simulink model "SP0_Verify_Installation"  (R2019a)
settings: Solver=VariableStepAuto  StartTime=0.0  StopTime=0.01  FixedStep=1e-5  RelTol=5e-6
libraries: ee_lib x3, fl_lib x2, nesl_utility x2

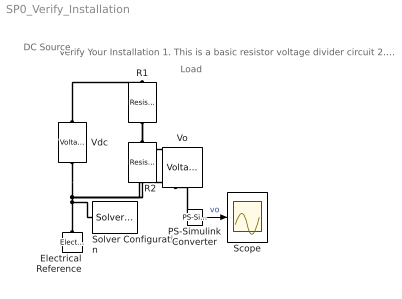
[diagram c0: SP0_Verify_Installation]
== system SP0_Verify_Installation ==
  note: Verify Your Installation 1. This is a basic resistor voltage divider circuit 2. Ensure you see a DC source and 2 resistors in the diagram 3. If you do not, you may have to re-install the Simscape Package 4. Simulate the circuit (click the Run button above) 5. Open the Scope below (double click) 6. Observe the voltage waveform 7. If you see a line at 5 V, your installation is correct, hurray! 8. If the simulation does not run, check with a classmate, TA, or Prof. Kim _________________________________
  note: Load
  note: DC Source
  Electrical Reference : fl_lib/Electrical/Electrical Elements/Electrical Reference
  PS-Simulink Converter : nesl_utility/PS-Simulink Converter  PhysicalDomain=network_engine_domain  SubClassName=ps_output  LeftPortType=input  RightPortType=output  PseudoPeriodic=off  Frequencies=[]  Unit=1  AffineConversion=off
  R1 : ee_lib/Passive/Resistor  R=5 Ohm  R_tol=1  enable_R_tol=0  tol_distribution=1  nSigma=4  enable_operating_limits=0  operating_limit_action=2  max_working_voltage=100 V  power_rating=1 W  enable_faults=0  fault_action=1  R_faulted=inf Ohm  enable_temporal_fault=0  t_fault=1 s  enable_behavioral_fault=0  max_permissible_current=1 A  t_fail_on_current=1 s  noise_mode=0  sample_time=1e-3 s  repeatability=1  auto_seed=1127352614  user_seed=0  Tdevice=25 degC  alpha=3.93e-3 1/K  Tmeas=25 degC  thermal_mass=100 J/K  power_derating_T1=70 degC  power_derating_T2=155 degC  operating_temperature_range_vec=[-50, 150] degC  temperature_specify=off  temperature_priority=High  temperature=298.15 K  temperature_nominal_specify=off  temperature_nominal_unit=K  temperature_nominal_value=1
  R2 : ee_lib/Passive/Resistor  R=5 Ohm  R_tol=1  enable_R_tol=0  tol_distribution=1  nSigma=4  enable_operating_limits=0  operating_limit_action=2  max_working_voltage=100 V  power_rating=1 W  enable_faults=0  fault_action=1  R_faulted=inf Ohm  enable_temporal_fault=0  t_fault=1 s  enable_behavioral_fault=0  max_permissible_current=1 A  t_fail_on_current=1 s  noise_mode=0  sample_time=1e-3 s  repeatability=1  auto_seed=529650792  user_seed=0  Tdevice=25 degC  alpha=3.93e-3 1/K  Tmeas=25 degC  thermal_mass=100 J/K  power_derating_T1=70 degC  power_derating_T2=155 degC  operating_temperature_range_vec=[-50, 150] degC  temperature_specify=off  temperature_priority=High  temperature=298.15 K  temperature_nominal_specify=off  temperature_nominal_unit=K  temperature_nominal_value=1
  Scope : Scope
  Solver Configuration : nesl_utility/Solver Configuration  PhysicalDomain=network_engine_domain  SubClassName=solver  LeftPortType=input  RightPortType=generic  Tones=[]  Harmonics=[]  SimulateNoise=off  Profile=off  UseLocalSampling=off  EnableSwitchedLinearOptims=on  FrequencyDomain=off  UseCCode=off  RelTol=0.001  AbsTol=1e-06  MinStep=1e-09  ToWorkspace=off  RevertToSquareIcSolve=off  NumHomotopyIterations=100  PhasorMode=off  PhasorModeNumHarmonics=1  DoDC=off  ResidualTolerance=1e-09  UseLocalSolver=off  LocalSolverChoice=NE_BACKWARD_EULER_ADVANCER  LocalSolverSampleTime=0.001  DoFixedCost=off  MaxNonlinIter=3  MaxModeIter=2  LinearAlgebra=auto  EquationFormulation=NE_TIME_EF  DelaysMemoryBudget=1024  AutomaticFiltering=on  FilteringTimeConstant=0.001  PartitionStorageMethod=AS_NEEDED  PartitionMemoryBudget=1024  PartitionMethod=ROBUST
  Vdc : ee_lib/Sources/Voltage Source  dc_voltage=10 V  ac_voltage=0 V  ac_shift=0 rad  ac_frequency=0 Hz  noise_mode=0  PSD=0 V^2/Hz  repeatability=1  auto_seed=3499211588  user_seed=0  sample_time=1e-3 s  i_specify=off  i_priority=None  i=0 A  i_nominal_specify=off  i_nominal_unit=A  i_nominal_value=1  v_specify=off  v_priority=None  v=0 V  v_nominal_specify=off  v_nominal_unit=V  v_nominal_value=1
  Vo : fl_lib/Electrical/Electrical Sensors/Voltage Sensor
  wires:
  PS-Simulink Converter/1 -> Scope/1  "vo"
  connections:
  Vdc/RConn1 -- Solver Configuration/RConn1 -- Electrical Reference/LConn1 -- R2/RConn1 -- Vo/RConn2
  Vdc/LConn1 -- R1/LConn1
  PS-Simulink Converter/LConn1 -- Vo/RConn1
  R1/RConn1 -- Vo/LConn1 -- R2/LConn1
